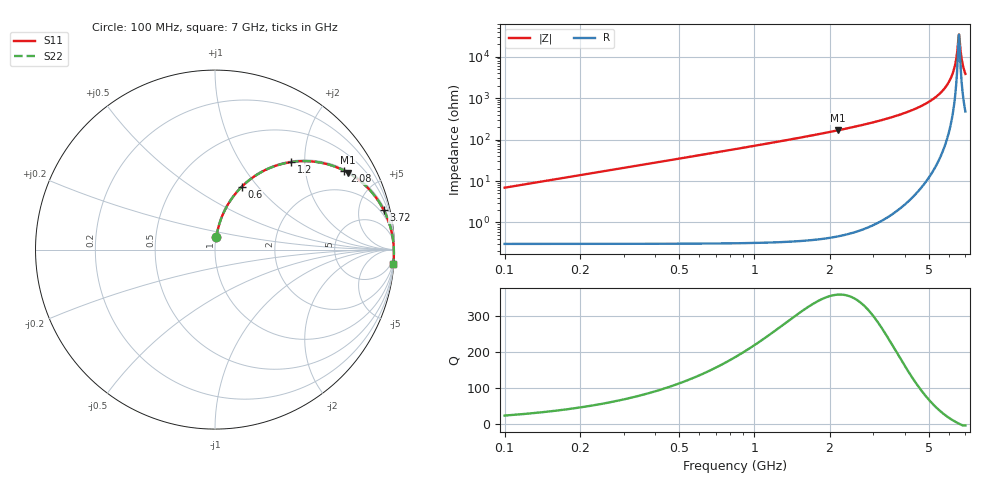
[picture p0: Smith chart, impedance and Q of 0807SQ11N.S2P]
! Coilcraft 0807SQ-11N Air Core Inductor
! 15 June 2010
# MHZ S MA R 50
!Freq  MagS11  AngS11  MagS21  AngS21  MagS12  AngS12  MagS22  AngS22
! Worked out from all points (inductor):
!   346 points, 100 MHz to 7 GHz, reference 50 ohm
!   read as one part in series: L = 11 nH near 120 MHz
!   highest Q = 361 at 2.16 GHz (marker M1), where L = 12.3 nH
!   self-resonance near 6.58 GHz
!   S11 on the Smith chart (normalised r, x): 100 MHz: 1.01, +0.14; 600 MHz: 1.01, +0.83; 1.2 GHz: 1.02, +1.71; 2.08 GHz: 1.06, +3.25; 3.72 GHz: 1.30, +8.37; 7 GHz: 1, -25
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100  0.06819 83.5  0.9947 -3.9  0.9947 -3.9  0.0682 83.5
180  0.1221 81.5  0.9895 -7.1  0.9895 -7.1  0.1221 81.5
280  0.1881 78.1  0.9792 -11.0  0.9792 -11.0  0.1881 78.1
600  0.3818 66.9  0.9214 -22.7  0.9214 -22.7  0.3818 66.9
1200  0.6465 49.0  0.7604 -40.8  0.7604 -40.8  0.6465 49.0
1260  0.666 47.5  0.7435 -42.3  0.7435 -42.3  0.666 47.5
2080  0.8444 31.3  0.5333 -58.5  0.5333 -58.5  0.8444 31.3
2160  0.8553 30.1  0.5157 -59.7  0.5157 -59.7  0.8554 30.1
2400  0.8835 26.7  0.4658 -63.1  0.4658 -63.1  0.8836 26.7
3560  0.9593 14.6  0.2781 -75.1  0.2781 -75.1  0.9593 14.6
3720  0.9649 13.3  0.2575 -76.4  0.2575 -76.4  0.965 13.3
4700  0.9869 6.6  0.1502 -82.8  0.1502 -82.8  0.987 6.6
5380  0.9939 2.8  0.08972 -85.9  0.08972 -85.9  0.9939 2.8
5860  0.9962 0.4  0.05196 -87.0  0.05196 -87.0  0.9963 0.4
6140  0.9969 -0.9  0.03149 -86.2  0.03149 -86.2  0.997 -0.9
6340  0.9971 -1.8  0.01754 -82.9  0.01754 -82.9  0.9972 -1.8
6460  0.9971 -2.3  0.009546 -75.3  0.009546 -75.3  0.9972 -2.3
6580  0.9971 -2.9  0.003091 -23.3  0.003091 -23.3  0.9971 -2.9
6600  0.9971 -2.9  0.002923 1.9  0.002923 1.9  0.9971 -2.9
6700  0.9969 -3.4  0.007442 62.9  0.007442 62.9  0.997 -3.4
6760  0.9969 -3.6  0.01113 70.5  0.01113 70.5  0.9969 -3.6
7000  0.9964 -4.6  0.02612 78.3  0.02612 78.3  0.9965 -4.6
